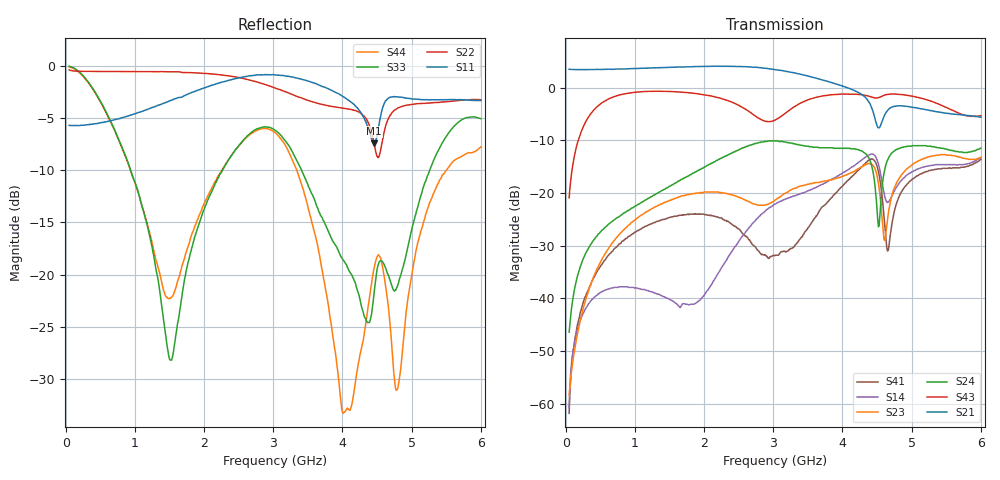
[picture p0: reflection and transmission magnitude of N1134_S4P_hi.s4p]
!S parameter
!Freq	Port1:RFIN1  Port2:RFOUT1  Port3:RFIN2  Port4:RFOUT2
# Hz S dB R 50
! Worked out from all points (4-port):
!   596 points, 50 MHz to 6 GHz, reference 50 ohm
!   strongest paths, dB at 50 MHz, 1.54 GHz, 3.03 GHz, 4.52 GHz, 6 GHz:
!     S21: 3.5, 3.9, 3.4, -7.6, -5.6
!     S43: -20.9, -0.7, -6.1, -1.9, -5.3
!     S24: -46.4, -18.4, -10.1, -26.4, -11.5
!     S23: -58.4, -21.2, -21.3, -18.2, -13.2
!     S14: -60.6, -40.4, -22.1, -14.5, -13.3
!     S41: -61.8, -24.5, -31.8, -15.9, -13.6
!   lowest |S11| = -7.4 dB at 4.46 GHz (marker M1), VSWR 2.48, Z = 29 + j28.9 ohm
!   |S11| at or under -10 dB: nowhere
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5e7  -5.71 179.0  -32.80 0.6  -73.90 15.8  -60.60 67.1
     3.51 -2.5  -0.39 -2.0  -58.40 106.0  -46.40 74.0
     -60.60 93.8  -59.60 83.8  -0.04 -5.2  -20.90 84.3
     -61.80 35.9  -65.70 -39.4  -20.90 84.3  -0.10 -5.7
6.1e8  -5.31 174.0  -35.90 7.0  -40.30 115.0  -38.20 47.2
       3.50 -22.6  -0.55 -12.4  -30.70 97.7  -26.00 57.1
       -46.30 51.8  -40.80 75.2  -4.77 -51.6  -2.20 32.5
       -31.90 76.5  -43.90 90.5  -2.20 32.5  -4.85 -56.1
2.17e9  -1.75 147.0  -19.20 121.0  -31.80 63.8  -36.00 134.0
        4.08 -93.5  -0.82 -62.5  -19.80 12.5  -13.90 3.6
        -28.90 120.0  -29.50 100.0  -11.20 63.8  -1.69 -29.6
        -24.50 -10.1  -34.60 -14.1  -1.77 -29.2  -11.00 9.4
3.27e9  -1.07 112.0  -10.80 79.2  -28.20 132.0  -20.70 109.0
        2.91 -167.0  -2.74 -131.0  -19.30 -25.1  -10.50 -82.8
        -27.80 103.0  -27.30 113.0  -8.17 -0.2  -4.27 -10.5
        -30.50 150.0  -34.10 -148.0  -3.91 -11.1  -8.95 -87.9
4.46e9  -7.44 106.0  -9.58 6.4  -12.70 56.2  -12.80 41.3
        -5.39 97.0  -7.57 135.0  -15.10 144.0  -17.50 165.0
        -12.30 56.7  -13.80 84.6  -21.60 98.8  -1.99 -48.3
        -13.80 44.1  -18.90 78.2  -1.92 -48.6  -19.30 86.7
4.62e9  -3.39 116.0  -14.50 28.0  -17.20 34.7  -21.10 31.3
        -4.91 126.0  -5.86 158.0  -28.40 170.0  -15.00 -119.0
        -16.60 28.5  -17.10 63.7  -19.30 88.5  -1.51 -49.5
        -27.40 11.3  -47.00 -79.6  -1.35 -49.7  -21.00 23.0
6e9  -3.33 102.0  -10.60 11.0  -15.50 30.1  -13.30 48.9
     -5.60 53.4  -3.26 111.0  -13.20 95.1  -11.50 132.0
     -16.10 32.7  -15.10 53.2  -5.07 116.0  -5.31 -83.1
     -13.60 60.5  -16.60 86.1  -5.31 -84.4  -7.77 169.0
